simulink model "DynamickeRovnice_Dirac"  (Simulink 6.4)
settings: Solver=ode45  StartTime=0.0  StopTime=4  MaxStep=1e-2  RelTol=1e-3

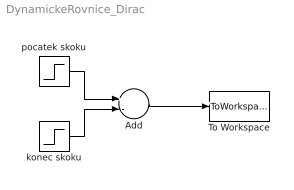
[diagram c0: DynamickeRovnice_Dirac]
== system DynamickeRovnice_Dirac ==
  Add : Sum  Inputs=+-  OutScaling=2^-10
  To Workspace : ToWorkspace  VariableName=dirac  SampleTime=-1  SaveFormat=Structure With Time
  konec skoku : Step  Time=3  After=0.5  SampleTime=0
  pocatek skoku : Step  After=0.5  SampleTime=0
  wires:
  Add/1 -> To Workspace/1
  pocatek skoku/1 -> Add/1
  konec skoku/1 -> Add/2
